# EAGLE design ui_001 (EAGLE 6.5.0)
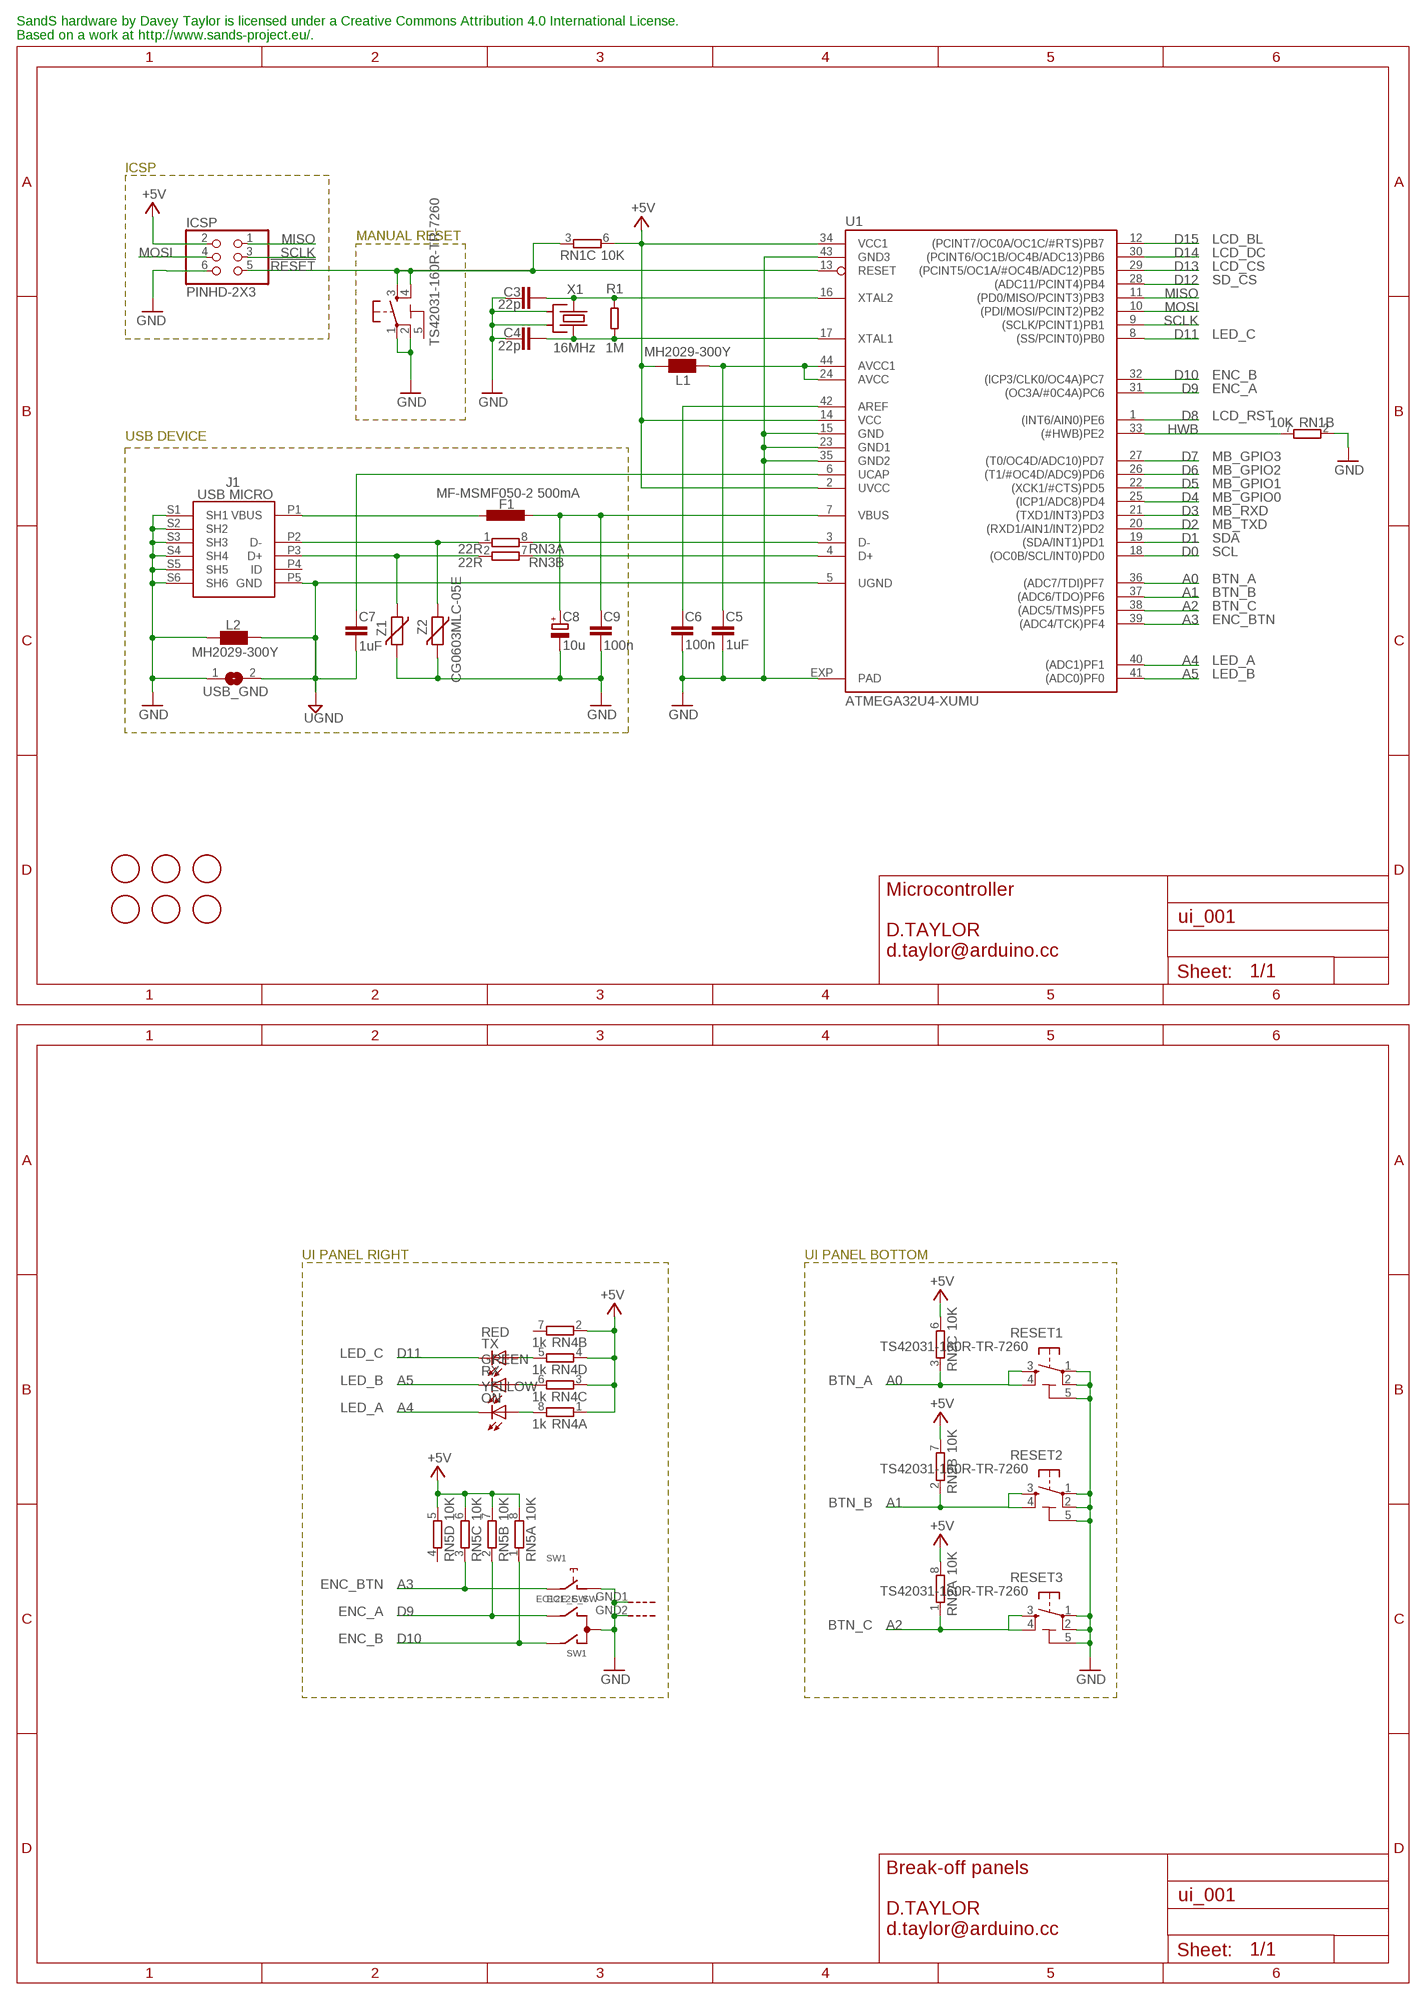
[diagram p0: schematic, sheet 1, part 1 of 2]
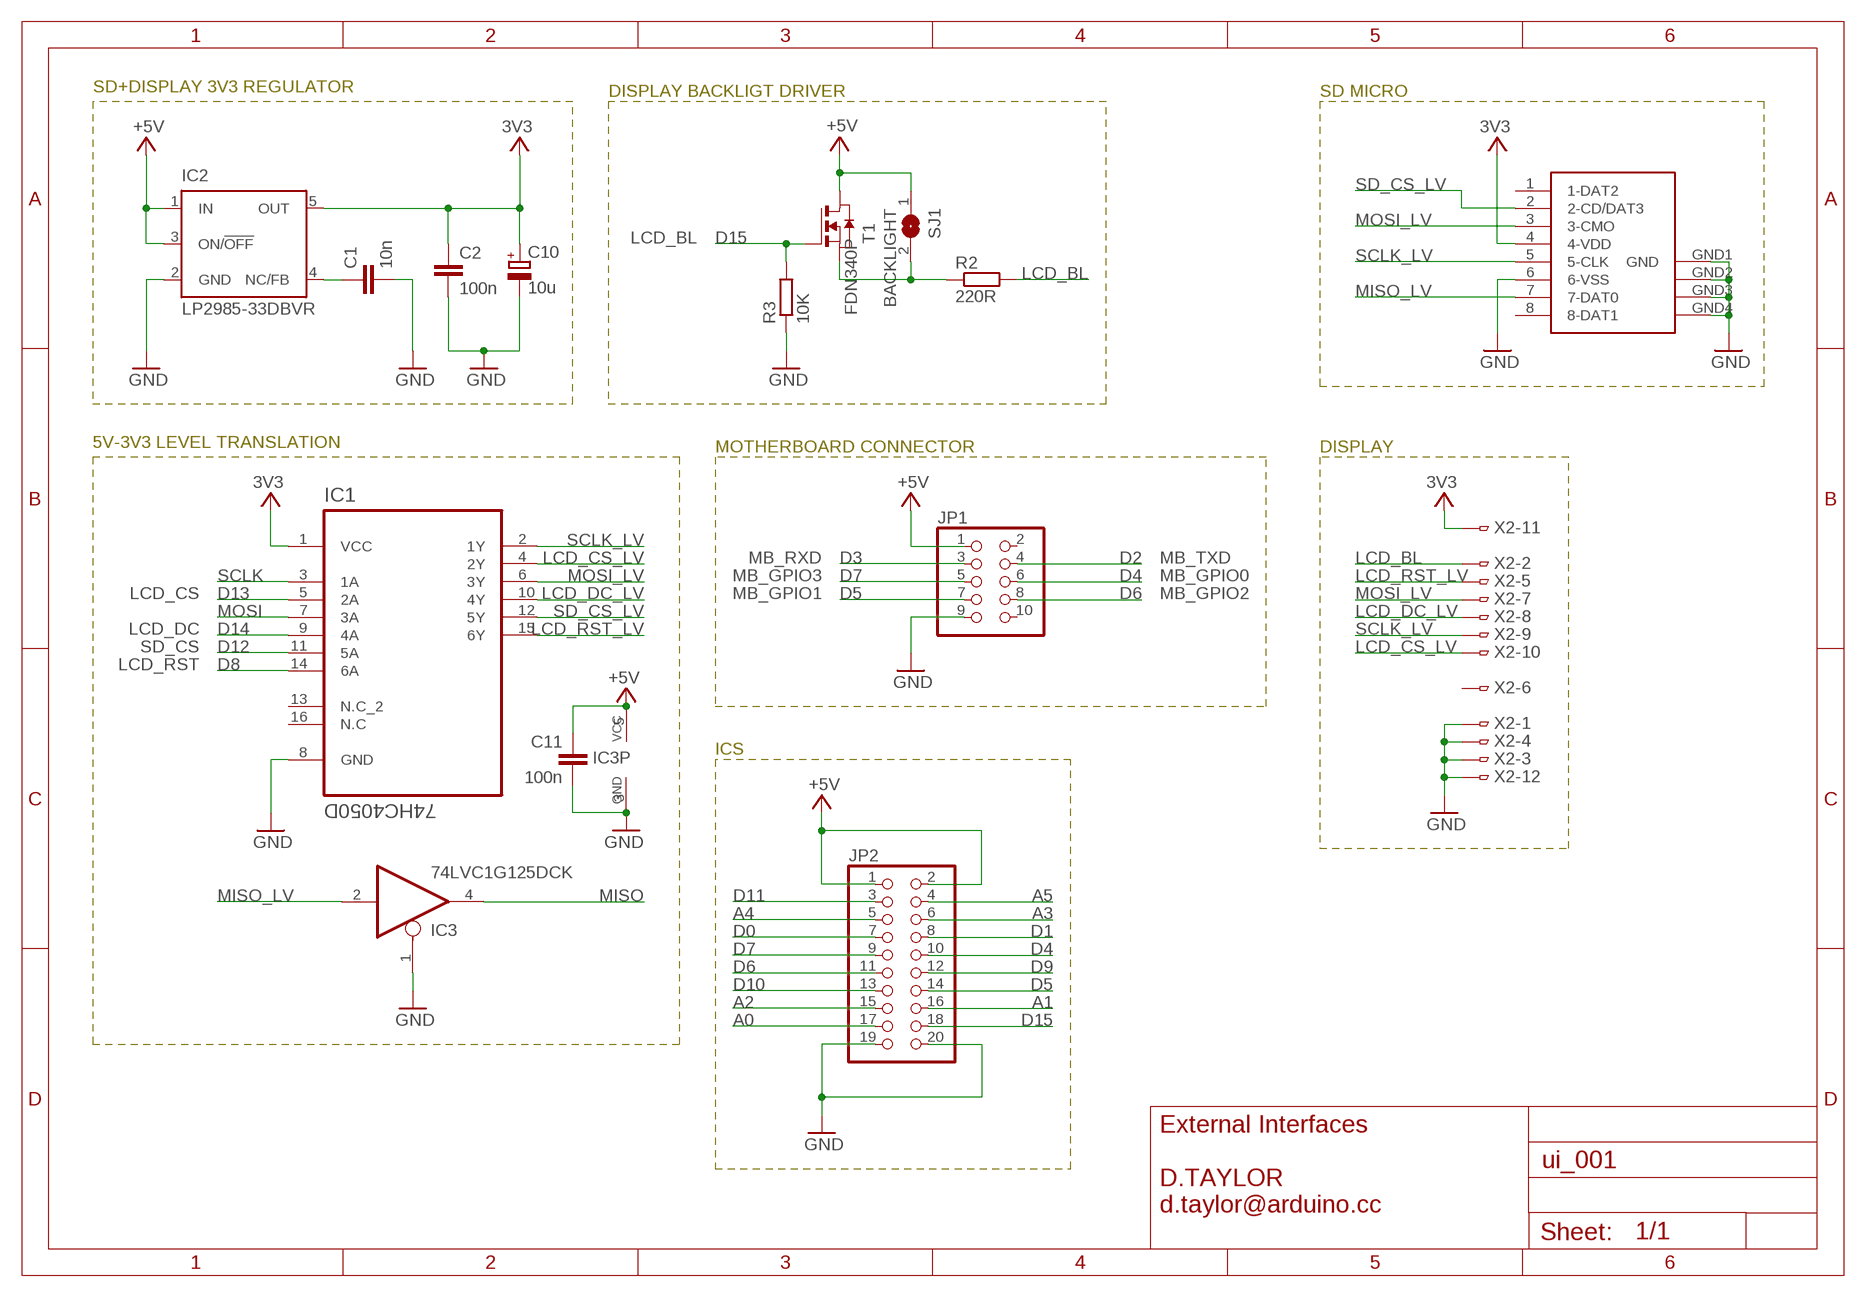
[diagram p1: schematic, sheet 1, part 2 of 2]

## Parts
C1  10n  C-EUC0603  [C0603-ROUND]
C2  100n  C-EUC0603  [C0603-ROUND]
C3  22p  C-EUC0603  [C0603-ROUND]
C4  22p  C-EUC0603  [C0603-ROUND]
C5  1uF  C-EUC0603  [C0603-ROUND]
C6  100n  C-EUC0603  [C0603-ROUND]
C7  1uF  C-EUC0603  [C0603-ROUND]
C8  10u  CPOL-EUSMCB  [SMC_B]
C9  100n  C-EUC0603  [C0603-ROUND]
C10  10u  CPOL-EUSMCB  [SMC_B]
C11  100n  C-EUC0603  [C0603-ROUND]
F1  MF-MSMF050-2 500mA  L-EUL1812  [L1812]
FID1  FIDUCIALMOUNT  [FIDUCIA-MOUNT]
FID2  FIDUCIALMOUNT  [FIDUCIA-MOUNT]
FID3  FIDUCIALMOUNT  [FIDUCIA-MOUNT]
FID4  FIDUCIALMOUNT  [FIDUCIA-MOUNT]
FID5  FIDUCIALMOUNT  [FIDUCIA-MOUNT]
FID6  FIDUCIALMOUNT  [FIDUCIA-MOUNT]
IC1  74HC4050D  [SOIC127P600X175-16N]
IC2  LP2985-33DBVR  LP2985-XXDBVR33  [SOT23-DBV]
IC3  74LVC1G125DCK  [SC70-5]
ICSP  PINHD-2X3  [2X03]
J1  USB MICRO  MYCON2_USB-MINI-B  [CON2_USB_MICRO_B_AT]
JP1  PINHD-2X5  [2X05]
JP2  PINHD-2X10  [2X10]
L1  MH2029-300Y  WE-CBF_0805  [0805]
L2  MH2029-300Y  WE-CBF_0805  [0805]
ON  YELLOW  LEDCHIPLED_0805  [CHIPLED_0805]
R1  1M  R-EU_0603-RND  [R0603-ROUND]
R2  220R  R-EU_0603-RND  [R0603-ROUND]
R3  10K  R-EU_0603-RND  [R0603-ROUND]
RESET  TS42031-160R-TR-7260  TS42  [TS42]
RESET1  TS42031-160R-TR-7260  TS42  [TS42]
RESET2  TS42031-160R-TR-7260  TS42  [TS42]
RESET3  TS42031-160R-TR-7260  TS42  [TS42]
RN1  10K  4R-NCAY16  [CAY16]
RN2  10K  4R-NCAY16  [CAY16]
RN3  22R  4R-NCAY16  [CAY16]
RN4  1k  4R-NCAY16  [CAY16]
RN5  10K  4R-NCAY16  [CAY16]
RX  GREEN  LEDCHIPLED_0805  [CHIPLED_0805]
SJ1  BACKLIGHT  SJ-NO  [SJ]
SW1  EC12E_SW  [ALPS_EC12E_SW]
T1  FDN340P  NMOSSOT23  [SOT-23]
TX  RED  LEDCHIPLED_0805  [CHIPLED_0805]
U1  ATMEGA32U4-XUMU  [QFN44ML7X7]
U2  SDCARD-15TW-8821  [SDCARD-15TW-8821]
USB_GND  SJ-NO  [SJ]
X1  16MHz  CRYSTAL2-KX7  [XTAL-3.2-2.5]
X2  FH12-12S-0.8SH  [FH12-12S-0.8SH]
Z1  CG0603MLC-05E  VARISTORCN0603  [CT/CN0603]
Z2  CG0603MLC-05E  VARISTORCN0603  [CT/CN0603]

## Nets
3V3: C2.1 C10.+ IC1.1(VCC) IC2.5(OUT) U2.4(4-VDD) X2.11
!RESET!: ICSP.5 RESET.3 RESET.4 RN1.3 U1.13(RESET)
+5V [usbvcc]: C11.1 IC2.1(IN) IC2.3(ON/!OFF) IC3.5(VCC) ICSP.2 JP1.1 JP2.1 JP2.2 L1.1 RN1.6 RN2.6 RN2.7 RN2.8 RN4.1 RN4.2 RN4.3 RN4.4 RN5.5 RN5.6 RN5.7 RN5.8 SJ1.1 T1.1(D) U1.2(UVCC) U1.14(VCC) U1.34(VCC1)
A0: JP2.17 RESET1.3 RESET1.4 RN2.3 U1.36((ADC7/TDI)PF7)
A1: JP2.16 RESET2.3 RESET2.4 RN2.2 U1.37((ADC6/TDO)PF6)
A2: JP2.15 RESET3.3 RESET3.4 RN2.1 U1.38((ADC5/TMS)PF5)
A3: JP2.6 RN5.3 SW1.E U1.39((ADC4/TCK)PF4)
A4: JP2.5 ON.C U1.40((ADC1)PF1)
A5: JP2.4 RX.C U1.41((ADC0)PF0)
AREF [aref]: C6.1 U1.42(AREF)
AVCC: C5.1 L1.2 U1.24(AVCC) U1.44(AVCC1)
D0: JP2.7 U1.18((OC0B/SCL/INT0)PD0)
D1: JP2.8 U1.19((SDA/INT1)PD1)
D2: JP1.4 U1.20((RXD1/AIN1/INT2)PD2)
D3: JP1.3 U1.21((TXD1/INT3)PD3)
D4: JP1.6 JP2.10 U1.25((ICP1/ADC8)PD4)
D5: JP1.7 JP2.14 U1.22((XCK1/#CTS)PD5)
D6: JP1.8 JP2.11 U1.26((T1/#OC4D/ADC9)PD6)
D7: JP1.5 JP2.9 U1.27((T0/OC4D/ADC10)PD7)
D8: IC1.14(6A) U1.1((INT6/AIN0)PE6)
D9: JP2.12 RN5.2 SW1.B U1.31((OC3A/#0C4A)PC6)
D10: JP2.13 RN5.1 SW1.A U1.32((ICP3/CLK0/OC4A)PC7)
D11: JP2.3 TX.C U1.8((SS/PCINT0)PB0)
D12: IC1.11(5A) U1.28((ADC11/PCINT4)PB4)
D13: IC1.5(2A) U1.29((PCINT5/OC1A/#OC4B/ADC12)PB5)
D14: IC1.9(4A) U1.30((PCINT6/OC1B/OC4B/ADC13)PB6)
D15: JP2.18 R3.2 T1.3(G) U1.12((PCINT7/OC0A/OC1C/#RTS)PB7)
D+: J1.P3(D+) RN3.2 Z1.1
D-: J1.P2(D-) RN3.1 Z2.1
GND [gnd]: C1.2 C2.2 C3.1 C4.2 C5.2 C6.2 C8.- C9.2 C10.- C11.2 IC1.8(GND) IC2.2(GND) IC3.1(OE) IC3.3(GND) ICSP.6 J1.S1(SH1) J1.S2(SH2) J1.S3(SH3) J1.S4(SH4) J1.S5(SH5) J1.S6(SH6) JP1.9 JP2.19 JP2.20 L2.2 R3.1 RESET1.1 RESET1.2 RESET1.5(5-GND) RESET2.1 RESET2.2 RESET2.5(5-GND) RESET3.1 RESET3.2 RESET3.5(5-GND) RESET.1 RESET.2 RN1.2 SW1.C SW1.D SW1.GND1(G) SW1.GND2(G) U1.15(GND) U1.23(GND1) U1.35(GND2) U1.43(GND3) U1.EXP(PAD) U2.6(6-VSS) U2.GND1(GND) U2.GND2(GND1) U2.GND3(GND2) U2.GND4(GND3) USB_GND.1 X1.2(SH1) X1.4(SH2) X2.1 X2.3 X2.4 X2.12 Z1.2 Z2.2
HWB: RN1.7 U1.33((#HWB)PE2)
LCD_BL: R2.2 X2.2
LCD_CS_LV: IC1.4(2Y) X2.10
LCD_DC_LV: IC1.10(4Y) X2.8
LCD_RST_LV: IC1.15(6Y) X2.5
MISO: IC3.4(O) ICSP.1 U1.11((PD0/MISO/PCINT3)PB3)
MISO_LV: IC3.2(I) U2.7(7-DAT0)
MOSI: IC1.7(3A) ICSP.4 U1.10((PDI/MOSI/PCINT2)PB2)
MOSI_LV: IC1.6(3Y) U2.3(3-CMO) X2.7
N$2: R2.1 SJ1.2 T1.2(S)
N$3: C1.1 IC2.4(NC/FB)
N$4: ON.A RN4.8
N$5: RN4.5 TX.A
N$6: RN4.6 RX.A
SCLK: IC1.3(1A) ICSP.3 U1.9((SCLK/PCINT1)PB1)
SCLK_LV: IC1.2(1Y) U2.5(5-CLK) X2.9
SD_CS_LV: IC1.12(5Y) U2.2(2-CD/DAT3)
UCAP: C7.1 U1.6(UCAP)
UGND [gnd]: C7.2 J1.P5(GND) L2.1 U1.5(UGND) USB_GND.2
USB_D+: RN3.7 U1.4(D+)
USB_D-: RN3.8 U1.3(D-)
USB_VCC: C8.+ C9.1 F1.1 U1.7(VBUS)
XTAL1: C4.1 R1.1 U1.17(XTAL1) X1.3(X2)
XTAL2: C3.2 R1.2 U1.16(XTAL2) X1.1(X1)
XUSB [usbvcc]: F1.2 J1.P1(VBUS)
Unconnected: IC1.13(N.C_2) IC1.16(N.C) J1.P4(ID) JP1.2 JP1.10 RN1.1 RN1.4 RN1.5 RN1.8 RN2.4 RN2.5 RN3.3 RN3.4 RN3.5 RN3.6 RN4.7 RN5.4 U2.1(1-DAT2) U2.8(8-DAT1) X2.6

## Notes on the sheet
- SandS hardware by Davey Taylor is licensed under a Creative Commons Attribution 4.0 International License.
  Based on a work at http://www.sands-project.eu/.
- ICSP
- MANUAL RESET | LCD_BL
- LCD_DC
- LCD_CS
- SD_CS
- LED_C
- ENC_B
- ENC_A
- LCD_RST
- USB DEVICE
- MB_GPIO3
- MB_GPIO2
- MB_GPIO1
- MB_GPIO0
- MB_RXD
- MB_TXD
- SDA
- SCL
- BTN_A
- BTN_B
- BTN_C
- ENC_BTN
- LED_A
- LED_B
- Microcontroller
  
  D.TAYLOR
  d.taylor@arduino.cc
- UI PANEL RIGHT | UI PANEL BOTTOM
- LED_C
- LED_B | BTN_A
- LED_A
- BTN_B
- ENC_BTN
- ENC_A
- BTN_C
- ENC_B
- Break-off panels
  
  D.TAYLOR
  d.taylor@arduino.cc
- SD+DISPLAY 3V3 REGULATOR | DISPLAY BACKLIGT DRIVER | SD MICRO
- LCD_BL
- 5V-3V3 LEVEL TRANSLATION | MOTHERBOARD CONNECTOR | DISPLAY
- MB_RXD | MB_TXD
- MB_GPIO3 | MB_GPIO0
- LCD_CS | MB_GPIO1 | MB_GPIO2
- LCD_DC
- SD_CS
- LCD_RST
- ICS
- External Interfaces
  
  D.TAYLOR
  d.taylor@arduino.cc

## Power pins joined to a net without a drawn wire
5-GND: RESET.5(5-GND)

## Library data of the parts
C1-C7 C9 C11 = SmartPrj:C-EU: CAPACITOR, European symbol
C8 = rcl:CPOL-EU: POLARIZED CAPACITOR, European symbol
C10 = SmartPrj:CPOL-EU: POLARIZED CAPACITOR, European symbol
F1 = rcl:L-EU: INDUCTOR, European symbol
FID1-FID6 = SmartPrj:FIDUCIALMOUNT
IC1 = SmartPrj:74HC4050D: Hex high-to-low level shifter; MPN: 74HC4050D; OC_FARNELL: 1085272; OC_NEWARK: -; PACKAGE: SOIC-16; SUPPLIER: NXP
IC2 = SmartPrj:LP2985-XXDBVR: ULTRALOW-POWER 50-mA LOW-DROPOUT LINEAR REGULATORS 50-mA Low-Dropout Regulator Source: http://focus.ti.com/lit/ds/symlink/tps77001.pdf
IC3 = 74xx-little-us:74*1G125: Single Bus Buffer Gate with 3-State Output
ICSP = SmartPrj:PINHD-2X3: PIN HEADER
J1 = d_taylor:MYCON2_USB-MINI-B
JP1 = pinhead:PINHD-2X5: PIN HEADER
JP2 = pinhead:PINHD-2X10: PIN HEADER
L1 L2 = wuerth-elektronik:WE-CBF: SMD EMI Suppression Ferrite Beads
ON RX TX = led:LED: LED
R1 = d_taylor:R-EU_: RESISTOR, European symbol
R2 R3 = SmartPrj:R-EU_: RESISTOR, European symbol
RESET RESET1-RESET3 = SmartPrj:TS42: TS42 Dongnan Electronics Tact switch VDC 12V - 50mA
RN1-RN5 = resistor-dil:4R-N: Array Chip Resistor Source: RS Component / Phycomp; OC_FARNELL: unknown; OC_NEWARK: unknown
SJ1 USB_GND = d_taylor:SJ?-NO: SMD solder JUMPER
SW1 = switch-alps:EC12E_SW: ALPS rotary Encoder EC12E series with switch; MPN: EC12E2424407; OC_FARNELL: 1520813; OC_NEWARK: 74M1068
T1 = zetex:NMOSSOT23: MOS FET; OC_FARNELL: unknown; OC_NEWARK: unknown
U1 = d_taylor:ATMEGA32U4-XU
U2 = st-mod v1.4:SDCARD-15TW-8821: SD Card SDCARD 15TW 8821
X1 = d_taylor:CRYSTAL2: KX7 SMD crystal
X2 = SmartPrj:FH12-12S-0.8S: 0.5mm Pitch Connectors For FPC/FFC Source: Data sheet; MPN: MC34827; OC_FARNELL: 1324544; OC_NEWARK: 41P0493
Z1 Z2 = varistor:VARISTOR: VARISTOR

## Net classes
0 default: width 0.203 mm, drill 0.406 mm, clearance 0.203 mm
2 gnd: width 0.203 mm, drill 0.406 mm, clearance 0.203 mm
3 usbvcc: width 0.203 mm, drill 0.406 mm, clearance 0.203 mm
4 aref: width 0.203 mm, drill 0.406 mm, clearance 0.203 mm

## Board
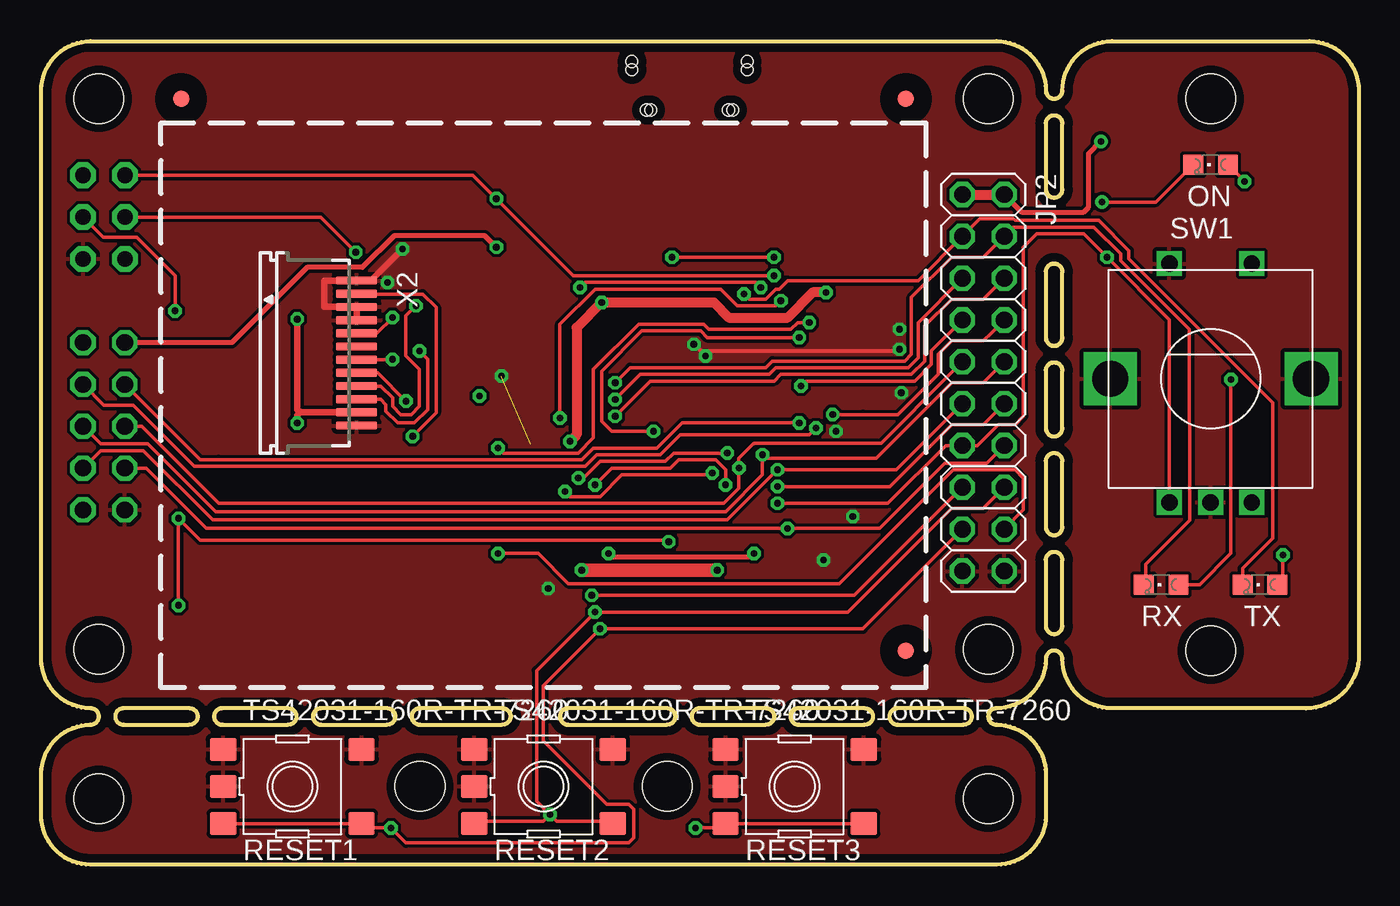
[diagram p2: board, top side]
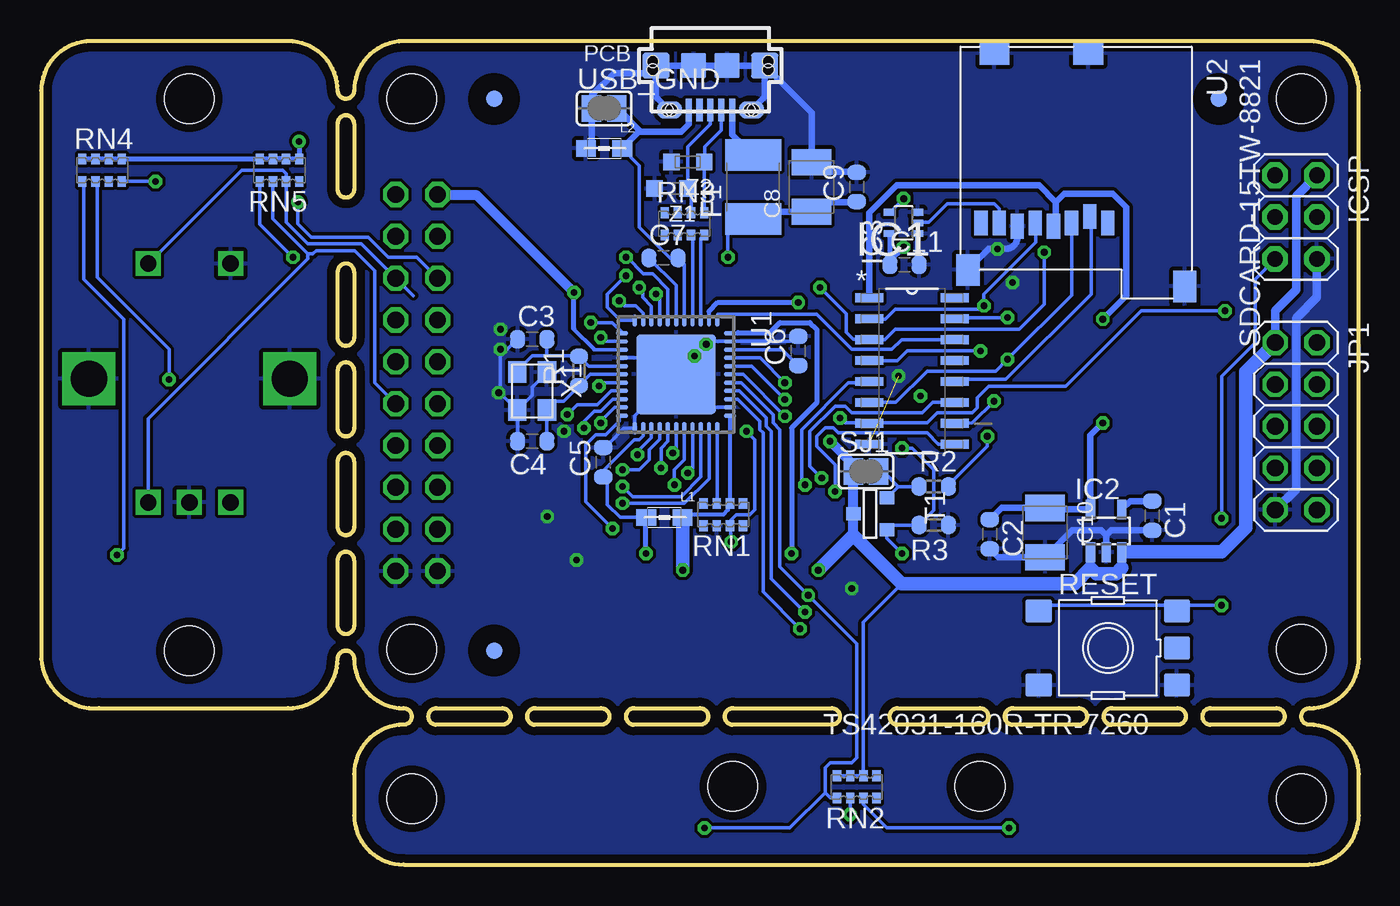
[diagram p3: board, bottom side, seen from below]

Size 80 x 50 mm. Coordinates in mm from the lower left corner, seen from the top.
Outline: 76 segments
Copper layers (1*16): Top 0.035mm / dielectric 1.5mm / Bottom 0.035mm
Design rules "default *": minimum track width 8mil, minimum drill 16mil, track to track 8mil, track to pad 8mil, pad to pad 8mil, via to via 8mil, smd to smd 8mil, copper to edge 20mil, drill to drill 8mil, minimum pad ring 10mil, minimum via ring 8mil, stop-mask expansion 4mil, vias tented up to drill 0mil, thermal gap 10mil
Holes 3 mm at 3.5,46.5 3.5,4 57.5,4 57.5,46.5 3.5,13.07 57.5,13.07 71,46.5 71,13 38,4.75 23,4.75

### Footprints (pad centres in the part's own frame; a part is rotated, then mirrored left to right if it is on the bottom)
C0603-ROUND = smd 0.898 x 1.1: 1 -0.889,0; 2 0.889,0
SMC_B = smd 1.6 x 2.4: + -1.5,0; - 1.5,0
L1812 = smd 1.9 x 3.4: 1 -1.95,0; 2 1.95,0
FIDUCIA-MOUNT = smd 1.016 x 1.016: P$1 0,0
SOIC127P600X175-16N = smd 1.702 x 0.533: 1 -2.591,4.445; 2 -2.591,3.175; 3 -2.591,1.905; 4 -2.591,0.635; 5 -2.591,-0.635; 6 -2.591,-1.905; 7 -2.591,-3.175; 8 -2.591,-4.445; 9 2.591,-4.445; 10 2.591,-3.175; 11 2.591,-1.905; 12 2.591,-0.635; 13 2.591,0.635; 14 2.591,1.905; 15 2.591,3.175; 16 2.591,4.445
SOT23-DBV = smd 0.55 x 1.2: 1 -0.95,-1.3; 2 0,-1.3; 3 0.95,-1.3; 4 0.95,1.3; 5 -0.95,1.3
SC70-5 = smd 0.4 x 0.7: 1 -0.65,-0.85; 2 0,-0.85; 3 0.65,-0.85; 4 0.65,0.85; 5 -0.65,0.85
2X03 = drill 0.95 pad 1.55 octagon: 1 -2.54,-1.27; 2 -2.54,1.27; 3 0,-1.27; 4 0,1.27; 5 2.54,-1.27; 6 2.54,1.27
CON2_USB_MICRO_B_AT = smd 0.406 x 1.346: P1 -1.321,2.692; P2 -0.66,2.692; P3 0,2.692; P4 0.66,2.692; P5 1.321,2.692 | smd 1.651 x 1.549: S1 -3.302,0; S2 3.302,0 | smd 1.524 x 1.016: S3 -2.489,2.692; S4 2.489,2.692 | smd 1.524 x 1.524: S5 -1.016,0; S6 1.016,0 | hole 0.7: -3.505,0.254; -3.505,-0.254; 3.505,0.254; 3.505,-0.254; -2.616,2.692; -2.362,2.692; 2.362,2.692; 2.616,2.692
2X05 = drill 1.016 octagon: 1 -5.08,-1.27; 2 -5.08,1.27; 3 -2.54,-1.27; 4 -2.54,1.27; 5 0,-1.27; 6 0,1.27; 7 2.54,-1.27; 8 2.54,1.27; 9 5.08,-1.27; 10 5.08,1.27
2X10 = drill 1.016 octagon: 1 -11.43,-1.27; 2 -11.43,1.27; 3 -8.89,-1.27; 4 -8.89,1.27; 5 -6.35,-1.27; 6 -6.35,1.27; 7 -3.81,-1.27; 8 -3.81,1.27; 9 -1.27,-1.27; 10 -1.27,1.27; 11 1.27,-1.27; 12 1.27,1.27; 13 3.81,-1.27; 14 3.81,1.27; 15 6.35,-1.27; 16 6.35,1.27; 17 8.89,-1.27; 18 8.89,1.27; 19 11.43,-1.27; 20 11.43,1.27
0805 = smd 1.2 x 1: 1 -1.1,0; 2 1.1,0
CHIPLED_0805 = smd 1.2 x 1.2: A 0,-1.05; C 0,1.05
R0603-ROUND = smd 0.898 x 1.1: 1 -0.889,0; 2 0.889,0
TS42 = smd 1.6 x 1.4: 1 -4.2,2.25; 2 4.2,2.25; 3 -4.2,-2.25; 4 4.2,-2.25; 5 -4.2,0
CAY16 = smd 0.5 x 0.65: 1 -1.2,-0.675; 2 -0.4,-0.675; 3 0.4,-0.675; 4 1.2,-0.675; 5 1.2,0.675; 6 0.4,0.675; 7 -0.4,0.675; 8 -1.2,0.675
SJ = smd 1.168 x 1.6: 1 -0.762,0; 2 0.762,0
ALPS_EC12E_SW = drill 1 square: A -2.5,-7.5; B 2.5,-7.5; C 0,-7.5; D -2.5,7; E 2.5,7 | drill 2.2 square: GND1 -6.1,0; GND2 6.1,0
SOT-23 = smd 0.787 x 0.889: 1 0.025,-1.016; 2 -0.94,1.016; 3 0.991,1.016
QFN44ML7X7 = smd 0.75 x 0.275: 1 -3.275,2.5; 2 -3.275,2; 3 -3.275,1.5; 4 -3.275,1; 5 -3.275,0.5; 6 -3.275,0; 7 -3.275,-0.5; 8 -3.275,-1; 9 -3.275,-1.5; 10 -3.275,-2; 11 -3.275,-2.5; 23 3.275,-2.5; 24 3.275,-2; 25 3.275,-1.5; 26 3.275,-1; 27 3.275,-0.5; 28 3.275,0; 29 3.275,0.5; 30 3.275,1; 31 3.275,1.5; 32 3.275,2; 33 3.275,2.5 | smd 0.275 x 0.75: 12 -2.5,-3.275; 13 -2,-3.275; 14 -1.5,-3.275; 15 -1,-3.275; 16 -0.5,-3.275; 17 0,-3.275; 18 0.5,-3.275; 19 1,-3.275; 20 1.5,-3.275; 21 2,-3.275; 22 2.5,-3.275; 34 2.5,3.275; 35 2,3.275; 36 1.5,3.275; 37 1,3.275; 38 0.5,3.275; 39 0,3.275; 40 -0.5,3.275; 41 -1,3.275; 42 -1.5,3.275; 43 -2,3.275; 44 -2.5,3.275 | smd 4.826 x 4.826: EXP 0,0
SDCARD-15TW-8821 = smd 0.8 x 1.5: 1 0,0; 2 1.1,-0.4; 3 2.2,0; 4 3.3,0.2; 5 4.4,0; 6 5.5,0.2; 7 6.6,0; 8 7.7,0 | smd 1.4 x 1.9: GND1 -4.66,3.85; GND2 8.49,2.85 | smd 1.8 x 1.4: GND3 1.19,-10.3; GND4 6.89,-10.3
XTAL-3.2-2.5 = smd 1.3 x 1.1: 1 -1.15,-0.9; 2 1.15,-0.9; 3 1.15,0.9; 4 -1.15,0.9
FH12-12S-0.8SH = smd 0.5 x 2.5: 1 -4.4,3.25; 2 -3.6,3.25; 3 -2.8,3.25; 4 -2,3.25; 5 -1.2,3.25; 6 -0.4,3.25; 7 0.4,3.25; 8 1.2,3.25; 9 2,3.25; 11 3.6,3.25; 12 4.4,3.25 | smd 0.55 x 2.5: 10 2.8,3.25
CT/CN0603 = smd 1 x 1: 1 -1,0; 2 1,0

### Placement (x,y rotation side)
C1  12.55,21.18 270 bottom
C2  22.4,20.07 270 bottom
C3  50.19,31.9 0 bottom
C4  50.19,25.7 180 bottom
C5  45.87,24.43 90 bottom
C6  34.04,31.19 90 bottom
C7  42.21,36.83 0 bottom
C8  33.22,41.15 90 bottom
C9  30.48,41.15 90 bottom
C10  19.05,20.17 270 bottom
C11  27.58,36.42 0 bottom
F1  36.78,41.15 90 bottom
FID1  52.5,13 0 bottom
FID2  8.5,46.5 0 bottom
FID3  52.5,46.5 0 bottom
FID4  8.5,46.5 0 top
FID5  52.5,46.5 0 top
FID6  52.5,13 0 top
IC1  27.13,29.97 0 bottom
IC2  15.34,20.27 0 bottom
IC3  27.64,38.96 90 bottom
ICSP  3.81,39.32 270 bottom
J1  39.37,48.51 180 bottom
JP1  3.81,26.62 270 bottom
JP2  57.2,29.26 270 top
L1  42.16,21.08 180 bottom
L2  45.82,43.48 180 bottom
ON  71,42.5 90 top
R1  47.35,29.97 90 bottom
R2  25.81,22.96 0 bottom
R3  25.81,20.62 180 bottom
RESET  15.24,13.16 180 bottom
RESET1  15.25,4.75 0 top
RESET2  30.5,4.75 0 top
RESET3  45.75,4.75 0 top
RN1  38.58,21.26 0 bottom
RN2  30.48,4.72 0 bottom
RN3  40.94,38.91 180 bottom
RN4  76.3,42.16 180 bottom
RN5  65.53,42.16 0 bottom
RX  68,17 90 top
SJ1  29.92,23.88 0 bottom
SW1  71,29.5 0 top
T1  29.67,21.34 270 bottom
TX  74,17 90 top
U1  41.45,29.77 270 bottom
U2  15.24,38.96 180 bottom
USB_GND  45.82,45.92 0 bottom
X1  50.19,28.75 270 bottom
X2  15.9,31.06 270 top
Z1  41.76,41.05 180 bottom
Z2  40.74,42.67 180 bottom

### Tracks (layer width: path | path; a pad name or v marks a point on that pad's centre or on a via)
3V3  (via drill 0.41)
  Top 0.406: X2.11 15.72,27.46 | 15.72,27.46 15.54,27.64 15.54,28.04 v15.54,33.12 | v15.54,26.82 15.54,27.29 15.72,27.46
  Bottom 0.203: 18.39,39.52 U2.4
  Bottom 0.406: v15.54,33.12 14.12,34.54 14.12,39.93 14.94,40.74 17.88,40.74 18.39,40.23 | 18.39,40.23 18.39,39.52 | IC1.1 29.72,39.57 28.04,41.25 19.41,41.25 18.39,40.23 | v15.54,26.82 16.29,26.08 IC2.5 18.95,21.57 C10.+ 21.69,21.67 C2.1
!RESET!  (via drill 0.41)
  Top 0.203: v8.33,15.75 8.33,19.71 v8.33,21.03 9.65,19.71 38,19.71 v38.1,19.61 38.2,19.71 | v37.19,26.31 34.65,26.31 34.04,26.92 34.04,29.97 36.47,32.41 40.03,32.41 40.44,32 v46.02,32
  Bottom 0.203: ICSP.5 6.3,35.56 6.3,31.7 8.33,29.67 v8.33,21.03 | RESET.3 10.69,15.75 v8.33,15.75 18.93,15.75 RESET.4 | v38.1,19.61 38.18,20.81 RN1.3 38.1,20.77 38.1,20.93 37.8,21.23 37.08,21.23 36.98,21.23 36.68,21.54 36.68,25.81 v37.19,26.31 | v46.02,32 45.79,31.77 U1.13
+5V  (via drill 0.41)
  Top 0.305: v27.64,37.49 26.92,38.2 22.25,38.2 21.44,38.2 19.51,36.27 16.15,36.27 11.58,31.7 JP1.1 | 46.84,34.75 v47.65,34.75 | JP2.2 59.54,39.62 63.3,39.62 63.6,39.93 63.6,43.18 v64.34,43.92
  Top 0.61: v32.11,25.7 32.51,26.11 32.51,32.61 v34.04,34.14 40.84,34.14 41.76,33.22 45.31,33.22 46.84,34.75 v47.65,34.75 | JP2.1 JP2.2
  Top 0.813: v41.05,17.88 v32.82,17.88
  Bottom 0.203: 41.05,21.26 L1.1 | 28.48,36.44 C11.1 28.45,36.7 | RN2.7 RN2.8 RN2.7 | RN2.7 RN2.6 30.08,5.89 30.07,5.89 30.07,14.73 27.74,17.07 | 38.28,21.66 38.28,21.86 RN1.6 38.18,22.04 | U1.14 46.41,31.27 46.43,31.29 | 65.91,42.86 65.91,42.93 RN5.7 | 65.15,42.86 65.15,42.93 RN5.6
  Bottom 0.254: 41.05,21.26 38.58,21.26 38.3,21.54 38.28,21.66 | U1.2 39.45,33.6 | 38.18,22.04 U1.34 | 46.43,31.29 47.65,32.51
  Bottom 0.305: IC3.5 28.48,36.44 | 28.45,36.7 v27.64,37.49 | 3.86,40.54 3.81,40.59 | 39.45,33.6 38.91,34.14 v34.04,34.14 | 30.68,24.28 SJ1.1 | 47.65,32.51 v47.65,34.75 | L1.1 41.06,20.85 41.05,20.83 | 65.15,42.86 65.91,42.86 | RN4.4 RN4.3 RN4.2 RN4.1 RN5.8 RN5.7 | v64.34,43.92 RN5.5 | RN5.5 | RN5.5 RN5.6
  Bottom 0.406: IC2.3 14.39,18.02 | IC2.1 16.29,18.02 | 30.68,23.24 SJ1.1 | 17.24,17.07 17.27,17.07
  Bottom 0.508: IC2.3 14.36,18.97 14.22,19 | JP1.1 5.08,33.63 3.81,34.9 3.81,40.59 ICSP.2
  Bottom 0.61: 30.68,23.24 T1.1 30.68,20.02 | v32.11,25.7 30.68,24.28 | v47.65,34.75 53.54,40.64 55.88,40.64 JP2.1
  Bottom 0.813: 14.39,18.02 14.73,17.68 15.95,17.68 16.29,18.02 17.24,17.07 | 14.22,19 8.33,19 6.86,20.47 6.86,29.92 JP1.1 | 17.27,17.07 27.74,17.07 30.68,20.02 v32.82,17.88 | 41.05,20.83 v41.05,17.88
A0  (via drill 0.41)
  Top 0.203: RESET1.3 RESET1.4 19.91,2.23 v21.23,2.23 22.15,1.32 35.66,1.32 35.97,1.63 35.97,3.35 35.66,3.66 34.34,3.66 30.48,7.52 30.48,10.87 v33.93,14.33 49.89,14.33 JP2.17
  Bottom 0.203: RN2.3 30.07,3.66 28.65,2.23 v21.23,2.23 | U1.36 37.72,28.27 36.37,26.92 36.37,26.42 36.17,26.21 36.17,25.81 36.17,16.56 v33.93,14.33
A1  (via drill 0.41)
  Top 0.203: v30.89,3.05 31.29,2.64 34.04,2.64 34.18,2.5 RESET2.4 | v30.89,3.05 30.48,2.64 26.92,2.64 26.78,2.5 RESET2.3 | JP2.16 57.2,21.64 55.27,21.64 48.97,15.34 v33.63,15.34 30.07,11.79 30.07,3.86 v30.89,3.05
  Bottom 0.203: RN2.2 30.88,3.21 v30.89,3.05 | U1.37 37.61,28.77 35.97,27.13 35.97,26.62 35.66,26.31 35.66,25.7 35.66,17.37 v33.63,15.34
A2  (via drill 0.41)
  Top 0.203: v39.73,2.23 41.35,2.23 RESET3.3 RESET3.4 | v33.43,16.36 49.38,16.36 JP2.15
  Bottom 0.203: 31.7,3.96 RN2.1 31.8,4.06 32.11,4.06 32.41,4.37 | v39.73,2.23 34.95,2.23 34.55,2.23 32.41,4.37 | U1.38 37.5,29.27 35.56,27.33 35.56,26.82 35.15,26.42 35.15,25.6 35.15,18.09 v33.43,16.36 30.48,13.41 30.48,6.5 30.79,6.2 32.11,6.2 32.41,5.89 32.41,4.37
A3  (via drill 0.41)
  Top 0.203: v34.85,27.23 36.98,29.36 44.5,29.36 44.91,29.77 52.73,29.77 52.83,29.77 53.65,30.58 53.65,32.72 55.27,34.34 57.2,34.34 JP2.6
  Bottom 0.203: U1.39 37.39,29.77 v34.85,27.23 | 57.4,34.54 58.42,35.56 JP2.6 60.55,37.69 63.8,37.69 65.13,39.02 RN5.3 65.13,41.96 65.33,42.16 67.84,42.16 SW1.E
A4  (via drill 0.41)
  Top 0.203: v34.85,28.25 36.37,29.77 44.2,29.77 44.6,30.18 52.63,30.18 53.24,30.79 53.24,32.92 JP2.5 | v64.41,40.23 67.68,40.23 ON.C
  Bottom 0.203: U1.40 36.87,30.27 v34.85,28.25 | JP2.5 57.2,36.88 58.93,36.88 60.15,38.1 63.6,38.1 64.41,38.91 v64.41,40.23
A5  (via drill 0.41)
  Top 0.203: v34.85,29.26 35.76,30.18 43.99,30.18 44.4,30.58 52.43,30.58 52.83,30.99 52.83,34.44 55.27,36.88 57.2,36.88 57.81,37.49 JP2.4 59.03,38.71 63.91,38.71 65.53,37.08 65.53,36.68 69.7,32.51 69.72,20.9 67.06,18.24 67.06,17.02 RX.C
  Bottom 0.203: U1.41 36.36,30.77 v34.85,29.26 | 58.55,38.23 JP2.4
AREF
  Bottom 0.203: U1.42 35,31.27 C6.1
AVCC  (via drill 0.41)
  Top 0.305: v34.44,18.9 34.65,18.69 43.08,18.69 v43.28,18.9
  Bottom 0.203: 43.45,21.08 L1.2 44.86,21.08 45.62,21.84 45.62,23.27 45.87,23.52 C5.1 45.82,23.98 43.99,25.81 43.69,25.81 43.46,26.04 U1.24
  Bottom 0.254: U1.44 37.73,32.27 37.69,32.31
  Bottom 0.305: 37.69,32.31 35.76,32.31 35.15,32.92 33.33,32.92 32.92,32.51 32.92,28.04 34.44,26.52 v34.44,18.9 | v43.28,18.9 43.28,21.06 L1.2
D0  (via drill 0.41)
  Top 0.203: v46.13,29.06 46.43,29.36 53.03,29.36 54.05,30.38 54.05,31.19 JP2.7
  Bottom 0.203: U1.18 45.91,29.27 v46.13,29.06
D1  (via drill 0.41)
  Top 0.203: v48.06,27.33 49.89,27.33 52.02,27.33 54.46,29.77 54.46,30.99 55.27,31.8 57.2,31.8 57.71,32.31 JP2.8
  Bottom 0.203: U1.19 45.4,28.77 46.23,27.94 47.45,27.94 v48.06,27.33
D2  (via drill 0.41)
  Top 0.203: JP1.4 3.81,27.89 5.59,27.89 9.3,24.18 10.77,24.18 33.02,24.18 33.73,24.89 37.59,24.89 38.81,26.11 46.63,26.11 v47.04,26.52
  Bottom 0.203: v47.04,26.52 47.04,26.92 46.43,27.53 46.02,27.53 45.29,28.27 U1.20
D3  (via drill 0.41)
  Top 0.203: v46.02,26.82 38.91,26.82 37.39,25.3 33.53,25.3 32.82,24.59 10.77,24.59 9.65,24.59 JP1.3
  Bottom 0.203: U1.21 45.18,27.77 46.02,26.92 v46.02,26.82
D4  (via drill 0.41)
  Top 0.203: JP1.6 3.61,25.55 6.48,25.55 10.59,21.44 10.77,21.44 36.47,21.44 41.55,21.44 43.79,23.67 v43.79,24.89 43.92,24.76 arc45 44.1,24.69 50.67,24.69 50.7,24.69 55.27,29.26 57.2,29.26 57.71,29.77 JP2.10
  Bottom 0.203: U1.25 42.95,25.93 43.69,25.2 43.79,25.09 v43.79,24.89
D5  (via drill 0.41)
  Top 0.203: JP1.7 6.38,24.08 10.03,20.42 10.77,20.42 v45.31,20.42 50.9,20.42 54.86,24.38 57.4,24.38 JP2.14
  Bottom 0.203: U1.22 44.91,27.27 44.91,26.93 | v45.31,20.42 46.94,22.05 46.94,25.5 46.33,26.11 45.72,26.11 44.91,26.92 | 44.91,26.92 arc-45 44.91,26.93 | 44.91,26.93 44.91,26.92 | 44.91,26.92 44.91,26.93
D6  (via drill 0.41)
  Top 0.203: JP1.8 3.61,25.15 6.2,25.15 10.41,20.93 11.3,20.93 | 10.77,20.93 11.3,20.93 | 11.3,20.93 36.58,20.93 41.66,20.93 v44.7,23.98 50.77,23.98 51.92,23.98 JP2.11
  Bottom 0.203: U1.26 42.45,25.82 43.08,25.2 43.08,24.59 43.69,23.98 v44.7,23.98
D7  (via drill 0.41)
  Top 0.203: JP1.5 6.1,26.62 10.77,21.95 36.37,21.95 41.45,21.95 42.37,22.86 v42.37,24.08 42.37,24.69 43.21,25.53 arc-45 43.39,25.6 51,25.6 55.17,29.77 JP2.9
  Bottom 0.203: U1.27 41.95,25.71 42.37,25.3 v42.37,24.08
D8
  Bottom 0.203: IC1.14 27.76,31.88 28.35,31.29 30.79,31.29 32.92,33.43 38.91,33.43 U1.1
D9  (via drill 0.41)
  Top 0.203: v44.7,22.96 51.51,22.96 55.27,26.72 57.2,26.72 JP2.12
  Bottom 0.203: U1.31 39.95,23.55 41.15,22.35 41.86,22.35 44.09,22.35 v44.7,22.96 | JP2.12 59.74,29.26 59.74,36.07 60.96,37.29 63.3,37.29 63.5,37.08 63.8,37.08 | 63.8,37.08 65.93,39.21 RN5.2 | SW1.B 73.5,27.08 63.8,36.78 63.8,37.08
D10  (via drill 0.41)
  Top 0.203: v44.7,21.95 51.41,21.95 54.91,25.45 JP2.13 56.84,25.45 58.12,26.72 59.13,26.72 59.64,27.23 59.64,37.49 60.45,38.3 63.3,38.3 v64.72,36.88 68.5,33.1 SW1.A
  Bottom 0.203: U1.32 39.45,23.44 40.95,21.95 42.16,21.95 44.91,21.95 v44.7,21.95 | v64.72,36.88 66.73,38.89 RN5.1
D11  (via drill 0.41)
  Top 0.203: v42.67,34.65 42.98,34.34 43.99,34.34 44.6,34.95 44.81,34.95 45.31,35.46 53.24,35.46 JP2.3 57,39.22 59.03,39.22 59.13,39.12 63.6,39.12 64.21,39.12 66.04,37.29 66.04,36.78 74.78,28.04 74.78,19.81 72.95,17.98 TX.C
  Bottom 0.203: U1.8 42.45,34.43 v42.67,34.65
D12  (via drill 0.41)
  Top 0.203: v41.66,24.99 38.41,24.99 37.9,24.49 33.93,24.49 32.92,23.47 v32.61,23.47
  Bottom 0.203: IC1.11 25.88,28.07 26.52,27.43 30.79,27.43 31.19,27.84 31.8,27.84 33.33,26.31 33.33,25.7 33.33,24.18 v32.61,23.47 | U1.28 41.45,25.2 v41.66,24.99
D13  (via drill 0.41)
  Top 0.203: v41.55,23.06 41.55,23.98 40.95,24.59 38.71,24.59 38.2,24.08 34.65,24.08 v33.63,23.06
  Bottom 0.203: IC1.5 30.1,29.34 30.18,29.26 30.99,29.26 33.83,26.42 33.83,24.38 33.83,23.27 v33.63,23.06 | U1.29 40.95,24.59 41.55,23.98 v41.55,23.06
D14  (via drill 0.41)
  Top 0.203: v31.8,22.66 32.11,22.35 33.93,22.35 35.26,23.67 40.64,23.67 v40.74,23.77
  Bottom 0.203: IC1.9 25.53,25.53 26.21,26.21 31.29,26.21 31.6,26.21 31.9,26.52 32.41,26.52 32.92,26.01 32.92,25.4 31.8,24.28 v31.8,22.66 | v40.74,23.77 40.45,24.06 U1.30
D15  (via drill 0.41)
  Top 0.203: v27.74,25.3 28.04,24.99 32.61,24.99 33.53,25.91 33.53,30.07 36.27,32.82 40.23,32.82 40.54,32.51 45.52,32.51 45.92,32.92 v46.63,32.92 | v27.74,18.9 30.18,18.9 32,17.07 48.46,17.07 55.37,23.98 59.13,23.98 59.64,23.47 59.64,21.54 JP2.18
  Bottom 0.203: T1.3 28.37,20.62 R3.2 25.81,21.51 25.81,23.98 27.13,25.3 v27.74,25.3 | T1.3 28.63,20.34 | U1.12 44.73,32.33 45.31,32.92 v46.63,32.92 | T1.3 28.65,19.81 v27.74,18.9
D+
  Bottom 0.203: J1.P3 39.37,44.96 40.74,43.59 40.74,41.06 | RN3.2 40.55,40.83
  Bottom 0.305: 40.74,41.06 Z1.1 40.55,40.83
D-
  Bottom 0.203: J1.P2 38.71,44.6 39.73,43.59 39.73,42.69 | Z2.1 39.74,39.69
  Bottom 0.305: 39.73,42.69 Z2.1 | 39.74,39.69 RN3.1
GND  (via drill 0.41)  (1 unrouted)
  Top 0.254: 40.03,31.19 v39.62,31.6 40.03,31.19 | 40.03,31.19 52.02,31.19 v52.12,31.29 | v40.34,30.89 40.03,31.19
  Top 0.406: 20.02,35.46 v21.95,37.39 | X2.1 17.18,35.46 17.18,33.86 X2.3 X2.4
  Bottom 0.203: U1.EXP v40.34,30.89 v39.62,31.6 39.45,31.77 U1.43 34.55,31.77 C6.2 | U1.35 39.45,27.77 U1.EXP | U1.EXP 43.95,27.27 U1.23 44.63,26.49 45.52,25.6 C5.2 | U1.15 42.45,30.77 U1.EXP | X1.4 50.19,29 50.19,28.5 X1.2 | C11.2 26.79,36.51 | C4.2 X1.2 | C3.1 51.1,31.9 52.02,30.99 52.12,30.89 52.12,28.63 X1.2
  Bottom 0.254: v52.12,31.29 52.12,30.99 52.02,30.99
  Bottom 0.305: 26.79,36.51 IC3.1
  Bottom 0.406: J1.S2 J1.S6 J1.S5 J1.S1 | J1.S1 36.07,46.63 J1.S3 | J1.S2 42.67,46.63 J1.S4 | J1.S2 43.13,48.06 45.21,48.06 46.53,46.74 USB_GND.1 46.58,43.82 L2.2 | J1.S1 33.22,45.67 C8.- 32.64,42.06 30.79,42.06 30.76,42.04 C9.2 | U2.6 20.74,38.09 arc90 21.44,37.39 v21.95,37.39 | v21.95,37.39 22.45,37.39 | 22.45,37.39 U2.GND2 | v21.95,37.39 22.45,37.39 | C1.2 12.9,20.32 15.04,20.32 15.34,20.02 | 15.34,20.02 IC2.2 | C2.2 21.89,18.67 C10.- 17.4,20.32 16.36,20.32 15.65,20.32 15.34,20.02
  Bottom 0.508: JP1.9 3.81,22.81 3.81,33.17 2.54,34.44 ICSP.6
  other vias: 47.5,18.5 30.78,16.76 27.94,29.67 21.03,35.36 52.12,32.51 48.26,26.31 52.22,28.65 49.28,21.13
  pour Top: 80,50 0,50 0,0 61,0 61,9.5 80,9.5
  pour Bottom: 80,50 0,50 0,0 61,0 61,9.5 80,9.5
HWB
  Bottom 0.203: U1.33 38.95,22.07 RN1.7
LCD_BL  (via drill 0.41)
  Top 0.203: X2.2 19.89,34.66 19.91,34.65 23.16,34.65 23.98,33.83 23.98,27.43 v22.55,26.01
  Bottom 0.203: v22.55,26.01 22.55,25.4 24.89,23.06 24.92,23.04 R2.2
LCD_CS_LV  (via drill 0.41)
  Top 0.203: X2.10 20.61,28.26 20.93,27.94 20.93,27.53 21.64,26.82 22.66,26.82 23.47,27.64 23.47,30.68 v22.96,31.19
  Bottom 0.203: IC1.4 28.02,30.61 27.43,31.19 v22.96,31.19
LCD_DC_LV  (via drill 0.41)
  Top 0.203: X2.8 20.42,29.87 v22.15,28.14
  Bottom 0.203: IC1.10 24,26.8 23.47,26.82 v22.15,28.14
LCD_RST_LV  (via drill 0.41)
  Top 0.203: X2.5 20.36,32.26 v21.34,33.22
  Bottom 0.203: IC1.15 24.41,33.15 24.38,33.12 23.88,33.22 v21.34,33.22
MISO  (via drill 0.41)
  Top 0.203: ICSP.1 26.21,41.86 v27.64,40.44 32.31,35.76 v44.5,35.76
  Bottom 0.203: v27.64,40.44 28.45,39.62 28.46,39.61 IC3.4 | v44.5,35.76 45.62,34.65 45.62,33.83 44.83,33.04 U1.11
MISO_LV
  Bottom 0.203: U2.7 21.84,39.82 22.15,40.13 24.99,40.13 26.11,39.01 26.73,39.01 IC3.2
MOSI  (via drill 0.41)
  Top 0.203: ICSP.4 3.76,38.1 5.79,38.1 8.13,35.76 v8.13,33.63 | v44.91,34.24 44.6,33.93 42.27,33.93 41.25,34.95 33.63,34.95 31.5,32.82 v31.5,27.13
  Bottom 0.203: 10.57,33.63 13.21,33.63 16.66,30.18 17.78,29.06 22.45,29.06 23.16,28.35 23.16,27.74 23.37,27.53 23.47,27.43 25.6,27.43 26.21,26.82 29.46,26.82 29.49,26.8 IC1.7 29.74,26.82 31.19,26.82 v31.5,27.13 | 10.57,33.63 v8.13,33.63 10.57,33.63 | U1.10 43.45,33.5 43.89,33.93 44.6,33.93 v44.91,34.24
MOSI_LV  (via drill 0.41)
  Top 0.203: X2.7 21.15,30.66 v21.34,30.68
  Bottom 0.203: IC1.6 28.12,28.07 26.21,29.97 22.05,29.97 v21.34,30.68 17.44,34.58 U2.3
N$1  (via drill 0.41)
  other vias: 26.62,28.45
N$2
  Bottom 0.203: R2.1 27.96,22.96 | 27.96,22.96 T1.2 | 27.96,22.96 28.88,23.88 SJ1.2
N$3
  Bottom 0.406: C1.1 13.88,22.07 IC2.4
N$4  (via drill 0.41)
  Top 0.203: v73.06,41.49 ON.A
  Bottom 0.203: RN4.8 v73.06,41.49
N$5  (via drill 0.41)
  Top 0.203: TX.A 75.22,17.17 75.29,17.17 75.39,17.27 v75.39,18.8
  Bottom 0.203: v75.39,18.8 74.98,19.2 74.98,33.12 77.42,35.56 77.42,41.35 RN4.5
N$6  (via drill 0.41)
  Top 0.203: v72.24,29.46 72.24,18.9 70.34,17 RX.A
  Bottom 0.203: v72.24,29.46 72.24,31.29 76.61,35.66 76.61,41.39 RN4.6
SCLK  (via drill 0.41)
  Top 0.203: v19.1,37.19 16.97,39.32 5.49,39.32 ICSP.3 | v32.72,35.05 33.02,35.36 43.38,35.36 v43.69,35.05
  Bottom 0.203: v19.1,37.19 19.1,34.04 20.62,32.51 22.35,32.51 28.14,32.51 28.78,31.88 IC1.3 29.79,31.8 30.48,31.9 30.68,31.9 31.11,32.33 31.11,33.45 v32.72,35.05 | U1.9 42.95,33.91 43.48,34.44 43.48,34.85 v43.69,35.05
SCLK_LV  (via drill 0.41)
  Top 0.203: X2.9 20.62,29.06 21.34,28.35 21.34,27.84 21.84,27.33 22.45,27.33 22.96,27.84 22.96,30.07 22.15,30.89 22.15,33.33 v22.76,33.93
  Bottom 0.203: IC1.2 29.72,33.07 29.67,33.12 28.75,33.12 28.14,33.73 22.96,33.73 v22.76,33.93 22.76,34.65 19.61,37.8 19.61,38.83 U2.5 19.64,39.59
SD_CS_LV
  Bottom 0.203: IC1.12 23.9,29.34 23.67,29.46 21.44,29.46 16.26,34.65 16.26,39.28 U2.2 | U2.2 16.34,39.64 16.46,39.52 | U2.2 16.52,39.97 16.56,39.93
UCAP
  Bottom 0.203: U1.6 41.45,35.18 C7.1
UGND
  Bottom 0.203: 43.69,44.4 43.59,44.5 | U1.5 40.95,36.46 C7.2 41.81,36.83 43.69,38.71 43.69,42.45 L2.1
  Bottom 0.406: J1.P5 40.69,44.96 41.15,44.5 43.59,44.5 43.69,44.6 | 43.69,44.6 45.01,45.92 USB_GND.2 | 43.69,44.6 43.69,44.52 L2.1
USB_D+
  Bottom 0.203: U1.4 40.45,38.04 RN3.7
USB_D-
  Bottom 0.203: U1.3 39.95,38.03 RN3.8
USB_VCC  (via drill 0.41)
  Top 0.203: v44.5,36.88 v38.3,36.88
  Bottom 0.203: v38.3,36.88 38.3,38.41 F1.1 | U1.7 41.95,34.94 42.88,35.87 42.9,35.89 43.43,35.89 44.42,36.88 v44.5,36.88
  Bottom 0.406: F1.1 36.33,39.65 C8.+ 32.64,40.23 30.79,40.23 30.76,40.26 C9.1
XTAL1
  Bottom 0.203: U1.17 46.66,29.77 R1.1 48.28,28.14 48.87,28.14 49.29,27.72 X1.3 49.3,27.59 C4.1
XTAL2
  Bottom 0.203: U1.16 46.75,30.27 R1.2 47.55,30.86 47.55,30.89 49.28,30.89 | 49.28,30.89 50.19,30.89 51.1,29.97 51.1,29.9 X1.1 | C3.2 49.3,30.91 49.28,30.89
XUSB
  Bottom 0.406: J1.P1 38.05,44.32 F1.2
